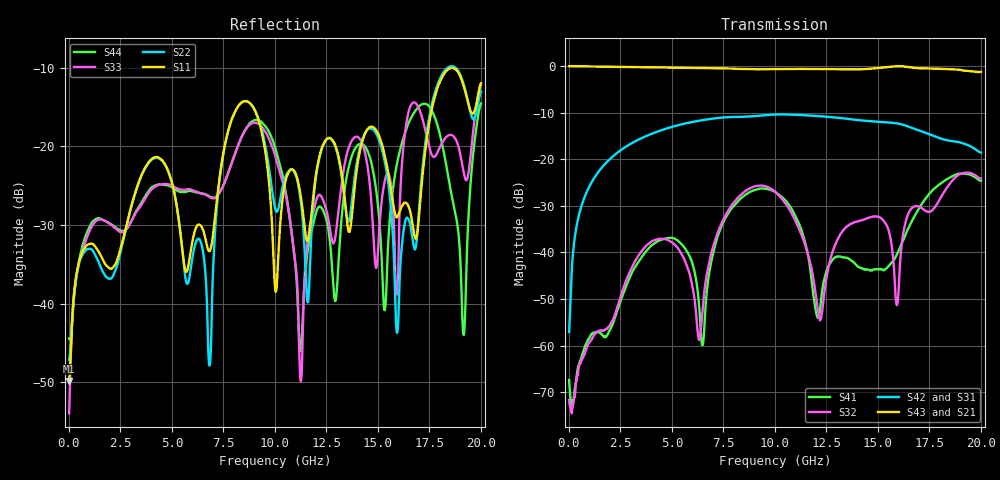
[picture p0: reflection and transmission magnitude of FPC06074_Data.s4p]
!Agilent Technologies,N5225A,MY51451324,A.10.20.03
!Agilent N5225A: A.10.20.03
!Date: Thursday, February 12, 2015 14:13:57
!Correction: S11(Full 4 Port(1,2,3,4))
!S12(Full 4 Port(1,2,3,4))
!S13(Full 4 Port(1,2,3,4))
!S14(Full 4 Port(1,2,3,4))
!S21(Full 4 Port(1,2,3,4))
!S22(Full 4 Port(1,2,3,4))
!S23(Full 4 Port(1,2,3,4))
!S24(Full 4 Port(1,2,3,4))
!S31(Full 4 Port(1,2,3,4))
!S32(Full 4 Port(1,2,3,4))
!S33(Full 4 Port(1,2,3,4))
!S34(Full 4 Port(1,2,3,4))
!S41(Full 4 Port(1,2,3,4))
!S42(Full 4 Port(1,2,3,4))
!S43(Full 4 Port(1,2,3,4))
!S44(Full 4 Port(1,2,3,4))
!S4P File: Measurements: <S11,S12,S13,S14>,
!<S21,S22,S23,S24>,
!<S31,S32,S33,S34>,
!<S41,S42,S43,S44>:
# Hz S  dB  R 50
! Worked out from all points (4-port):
!   2000 points, 10 MHz to 20 GHz, reference 50 ohm
!   strongest paths, dB at 10 MHz, 5.01 GHz, 10.01 GHz, 15.01 GHz, 20 GHz:
!     S43: 0.0, -0.3, -0.7, -0.4, -1.2
!     S21: 0.0, -0.3, -0.6, -0.5, -0.7
!     S42: -57.1, -13.0, -10.4, -12.0, -18.6
!     S31: -52.9, -13.0, -10.3, -12.0, -18.3
!     S32: -71.7, -37.8, -27.0, -32.3, -24.2
!     S41: -67.4, -36.9, -27.0, -43.6, -24.6
!   lowest |S11| = -49.9 dB at 10 MHz (marker M1), VSWR 1.01, Z = 49.8 + j0.283 ohm
!   |S11| at or under -10 dB: start of sweep to end of sweep
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1e7  -49.85 118.1  -0.03 -0.7  -56.67 107.6  -63.94 110.1
     -0.04 -0.8  -47.13 129.9  -63.30 174.9  -56.59 136.1
     -52.86 75.9  -71.66 41.7  -53.95 2.9  -0.03 -0.7
     -67.37 60.3  -57.05 2.0  -0.03 -0.8  -44.43 142.4
1.93e9  -35.43 18.9  -0.13 -34.4  -20.20 55.9  -57.45 151.2
        -0.14 -34.4  -36.83 51.1  -55.97 162.0  -20.22 54.8
        -20.21 55.9  -55.99 161.7  -29.77 45.4  -0.15 -34.9
        -57.06 151.3  -20.22 54.8  -0.15 -34.9  -29.74 48.6
1.028e10  -29.14 87.5  -0.61 -179.0  -10.35 -86.6  -27.90 -80.1
          -0.62 -178.9  -26.45 43.8  -28.21 -84.8  -10.40 -92.6
          -10.34 -86.5  -28.18 -84.9  -23.69 -86.4  -0.64 178.8
          -27.88 -80.0  -10.38 -92.6  -0.64 178.8  -22.70 -68.8
1.22e10  -20.90 -132.7  -0.61 146.9  -10.70 -120.3  -51.56 -58.7
         -0.61 147.1  -21.05 -128.1  -54.45 100.8  -10.78 -128.1
         -10.68 -120.2  -54.39 100.4  -26.22 65.4  -0.65 143.9
         -51.77 -57.5  -10.76 -128.1  -0.65 143.9  -27.67 46.1
1.593e10  -29.04 74.0  -0.40 77.5  -12.63 172.2  -40.40 91.4
          -0.41 77.7  -43.72 97.1  -51.89 -125.9  -12.31 160.9
          -12.63 172.3  -51.29 -126.4  -38.71 119.8  -0.05 74.7
          -40.34 91.2  -12.31 160.9  -0.05 74.7  -22.16 -4.3
1.916e10  -12.30 -62.2  -0.65 19.8  -16.16 119.4  -23.12 -64.3
          -0.64 20.0  -12.09 -63.9  -22.99 -60.0  -16.68 102.2
          -16.14 119.5  -22.97 -60.0  -23.24 -52.4  -0.98 15.6
          -23.08 -64.2  -16.65 102.1  -0.97 15.6  -43.95 -47.8
2e10  -12.00 31.6  -0.74 4.0  -18.34 99.9  -24.64 -101.2
      -0.73 4.2  -13.05 36.2  -24.15 -100.1  -18.58 81.2
      -18.32 100.1  -24.16 -100.2  -12.07 39.4  -1.25 2.3
      -24.63 -101.0  -18.56 81.2  -1.25 2.3  -14.57 45.2
